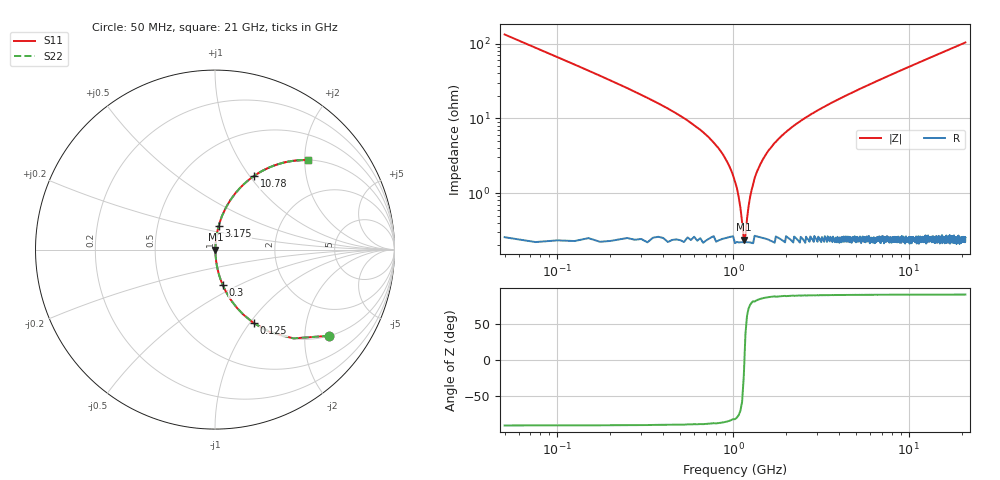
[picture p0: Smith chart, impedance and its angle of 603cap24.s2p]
! AVX Thin Film Operation		Date: November 2004
! Description: Accu-P® Series, Thin Film, SMD, RF Capacitor
! Part Number: 06033J240FBT
! 50 MHz  -  10.05 GHz
! Serial Measurements
# MHZ S MA R 50
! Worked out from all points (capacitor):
!   839 points, 50 MHz to 21 GHz, reference 50 ohm
!   read as one part in series: C = 24 pF near 150 MHz
!   lowest |Z| = 237 mohm at 1.15 GHz (marker M1)
!   series resonance near 1.159 GHz, so ESL is about 790 pH
!   S11 on the Smith chart (normalised r, x): 50 MHz: 1.01, -2.65; 125 MHz: 1.00, -1.05; 300 MHz: 1.00, -0.41; 3.175 GHz: 1.00, +0.27; 10.78 GHz: 1.00, +1.05; 21 GHz: 1.00, +2.07
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50  0.797 -37.0  0.602 52.9  0.602 52.9  0.797 -37.0
125  0.464 -62.1  0.884 27.6  0.884 27.6  0.464 -62.1
200  0.306 -71.8  0.95 17.8  0.95 17.8  0.306 -71.8
300  0.202 -77.7  0.977 11.6  0.977 11.6  0.202 -77.7
525  0.1 -82.9  0.993 5.7  0.993 5.7  0.1 -82.9
875  0.033 -83.9  0.997 1.9  0.997 1.9  0.033 -83.9
975  0.02 -82.0  0.997 1.1  0.997 1.1  0.02 -82.0
1100  0.006423 -67.7  0.998 0.3  0.998 0.3  0.006423 -67.7
1150  0.002556 -20.1  0.998 0.1  0.998 0.1  0.002556 -20.1
1225  0.006774 68.9  0.998 -0.4  0.998 -0.4  0.006774 68.9
1325  0.016 80.2  0.997 -0.9  0.997 -0.9  0.016 80.2
1425  0.024 82.9  0.997 -1.4  0.997 -1.4  0.024 82.9
1700  0.045 84.4  0.997 -2.6  0.997 -2.6  0.045 84.4
2275  0.083 83.6  0.994 -4.7  0.994 -4.7  0.083 83.6
3175  0.134 81.3  0.989 -7.7  0.989 -7.7  0.134 81.3
3550  0.154 80.2  0.986 -8.9  0.986 -8.9  0.154 80.2
7050  0.32 70.9  0.945 -18.7  0.945 -18.7  0.32 70.9
10525  0.456 62.6  0.888 -27.1  0.888 -27.1  0.456 62.6
10775  0.465 62.1  0.883 -27.7  0.883 -27.7  0.465 62.1
14025  0.566 55.3  0.823 -34.5  0.823 -34.5  0.566 55.3
17525  0.652 49.2  0.757 -40.7  0.757 -40.7  0.652 49.2
21000  0.718 44.0  0.694 -45.9  0.694 -45.9  0.718 44.0
